FUNCTION_BLOCK FB_IEDClient IMPLEMENTS I_ScsmAbortIndEventSink, I_ScsmGetServerDirectoryCnfEventSink, I_ScsmGetLogicalDeviceDirectoryCnfEventSink, I_ScsmGetLogicalNodeDirectoryCnfEventSink, I_ScsmGetDataValuesCnfEventSink, I_ScsmSetDataValuesCnfEventSink, I_ScsmReportIndEventSink, I_ScsmControlCnfEventSink, I_ScsmLastApplErrorIndEventSink, I_ScsmCommandTerminationIndEventSink
VAR_INPUT
	fbConnection		: FB_iec61850ClientClass := (ipAbortInd:=THIS^, ipGetServerDirectoryCnf:=THIS^, ipGetLogicalDeviceDirectoryCnf:=THIS^, ipGetLogicalNodeDirectoryCnf:=THIS^, ipGetDataValuesCnf:=THIS^, ipSetDataValuesCnf:=THIS^, ipReportInd:=THIS^, ipControlCnf:=THIS^, ipLastApplErrorInd:=THIS^, ipCommandTerminationInd:=THIS^);
END_VAR
VAR
	_bAbort				: BOOL; (* Rising edge activates AbortReq() command execution *)
	_bDisconnect		: BOOL; (* Rising edge activates ReleaseReq() command execution *)
	_bConnect			: BOOL; (* Rising edge activates AssociateReq() command execution *)
	_bReconnect			: BOOL := TRUE; (* TRUE => reconnect automatically *)
	_bReadAllData		: BOOL := TRUE; (* TRUE => read/refresh all data values on reconnect *)
	
	state				: BYTE;
	eState				: E_AsyncEnvironmentState; (* Environment state *)
	bBusy				: BOOL; (* If TRUE => command execution is busy *)
	bSuccess			: BOOL;
	ipResult			: I_AsyncServiceResultClass;
	sLastErrorResult	: T_MaxString;
	fbAbortReason		: FB_ServiceErrorClass := (stError:=SUCCESS_EVENT);
	sLastAbortReason	: T_MaxString;
	nInvokeID			: UDINT;
	eServiceError		: E_AcsiServiceError; (* Latest OnXyzCnf() or OnXyzInd() event handler error *)
	nServiceError		: UDINT; (* Counts OnXyzCnf() and OnXyzInd() event handler errors *)
	nCmdError			: UDINT; (* Counts xyzReq() command errors *)
	sObjReference		: T_AcsiObjectReference; (* DATA object reference *)
	sCtrlReference		: T_AcsiObjectReference; (* CONTROLLABLE-DATA object reference *)
	
	bGetServerDirectory				: BOOL := TRUE; (* Rising edge enumerates logical-devices *)
	bGetLogicalDeviceDirectory		: BOOL := TRUE; (* Rising edge enumerates logical-nodes *)
	bGetLogicalNodeDirectory		: BOOL := TRUE; (* Rising edge enumerates "IEDLD1/LLN0" data-sets *)
	bGetAllServerValues				: BOOL := TRUE; (* Rising edge reads all "IEDLD1" data attribute values *)
	bGetAllDataValues_LLN0_ST		: BOOL := TRUE; (* Rising edge reads all "IEDLD1/LLN0.ST" data attribute values (having selected functional constraint) *)
	bGetDataValues_LLN0_ST_Beh		: BOOL := TRUE; (* Rising edge reads all "IEDLD1/LLN0.ST.Beh" data attribute values (having selected functional constraint) *)

	bGetDataSetValues_LLN0_DS1		: BOOL := TRUE; (* Rising edge reads all member values of data-set: "IEDLD1/LLN0.DS1" *)
	bGetDataSetValues_LLN0_DS2		: BOOL := TRUE; (* Rising edge reads all member values of data-set: "IEDLD1/LLN0.DS2" *)
	bGetDataSetValues_LLN0_DS3		: BOOL := TRUE; (* Rising edge reads all member values of data-set: "IEDLD1/LLN0.DS3" *)
	bGetDataSetValues_LLN0_DS4		: BOOL := TRUE; (* Rising edge reads all member values of data-set: "IEDLD1/LLN0.DS4" *)
	bGetDataSetValues_LLN0_DS5		: BOOL := TRUE; (* Rising edge reads all member values of data-set: "IEDLD1/LLN0.DS5" *)
	bGetDataSetValues_LLN0_DS6		: BOOL := TRUE; (* Rising edge reads all member values of data-set: "IEDLD1/LLN0.DS6" *)
	bGetDataSetValues_LLN0_DS7		: BOOL := TRUE; (* Rising edge reads all member values of data-set: "IEDLD1/LLN0.DS7" *)
	bGetDataSetValues_LLN0_DS8		: BOOL := TRUE; (* Rising edge reads all member values of data-set: "IEDLD1/LLN0.DS8" *)

	bSetDataSetValues_LLN0_DS8		: BOOL := TRUE; (* Rising edge writes all member values of data-set: "IEDLD1/LLN0.DS8" *)
	
	sVendor 						: T_MaxString := 'MyCompany';
	sHwRev							: T_MaxString := '1.0';
	sSwRev 							: T_MaxString := '1.0';
	sSerNum							: T_MaxString := '123456';
	sModel							: T_MaxString := 'My61850Model';
	sLocation						: T_MaxString := 'MyLocation';
	sConfigRev						: T_MaxString := '1';
	nRev							: UDINT:=0;
END_VAR

fbConnection.Execute();
eState:= fbConnection.eState;

CASE state OF
	0: (* Initial state *)
		IF _bAbort THEN (* Abort connection => execute AbortReq() command *)
			_bAbort:= FALSE;
			bSuccess:= fbConnection.AbortReq(ipReason:=fbAbortReason, ipSink:=0, ipResult=>ipResult);
			state:= SEL(bSuccess, 100, 1);
		ELSIF eState = E_AsyncEnvironmentState.Idle AND (_bConnect OR _bReconnect) THEN (* Open/establish connection => execute AssociateReq() command *)
			_bConnect:= FALSE;
			bGetAllServerValues:= SEL(_bReadAllData, bGetAllServerValues, TRUE);
			bSuccess:= fbConnection.AssociateReq(ipSink:=0, ipResult=>ipResult);
			state:= SEL(bSuccess, 100, 1);
		ELSIF eState = E_AsyncEnvironmentState.Established AND _bDisconnect THEN (* Close/release connection => execute ReleaseReq() command *)
			_bDisconnect:= FALSE;
			bSuccess:= fbConnection.ReleaseReq(ipSink:=0, ipResult=>ipResult);
			state:= SEL(bSuccess, 100, 1);
		ELSIF eState = E_AsyncEnvironmentState.Established THEN (* Connection established => exchange IED data *)
			state:= 10;
		END_IF
		_bConnect:= FALSE;
		_bDisconnect:= FALSE;
		(*==================================================================================================================================================================*)
	1: (* Wait for AbortReq() or ReleaseReq() or AssociateReq() command completion *)
		IF ipResult <> 0 THEN
			ipResult.Execute();
			IF NOT (bBusy:=ipResult.IsBusy()) THEN
				state:= SEL(ipResult.IsCompleted(), 100(* failed or aborted *), 0(* succeeded *));
			END_IF
		END_IF
		(*==================================================================================================================================================================*)
	10: (* Read/Write IED data *)
		IF bGetServerDirectory THEN (* Example => execute GetServerDirectoryReq() command *)
			bGetServerDirectory:= FALSE;
			bSuccess:= fbConnection.GetServerDirectoryReq(ipServer:=fbIED, eClass:=E_AcsiServerDirectoryClass.LogicalDevice, hUser:=0, ipSink:=0, nInvokeID=>nInvokeID, ipResult=>ipResult);
			state:= SEL(bSuccess, 100, 11);
		ELSIF bGetLogicalDeviceDirectory THEN (* Example => execute GetLogicalDeviceDirectoryReq() command *)
			bGetLogicalDeviceDirectory:= FALSE;
			bSuccess:= fbConnection.GetLogicalDeviceDirectoryReq(ipLogicalDevice:=fbIED.IEDLD1, hUser:=0, ipSink:=0, nInvokeID=>nInvokeID, ipResult=>ipResult);
			state:= SEL(bSuccess, 100, 11);
		ELSIF bGetLogicalNodeDirectory THEN (* Example => execute GetLogicalNodeDirectoryReq() command *)
			bGetLogicalNodeDirectory:= FALSE;
			bSuccess:= fbConnection.GetLogicalNodeDirectoryReq(ipLogicalNode:=fbIED.IEDLD1.LLN0, eClass:=E_AcsiLogicalNodeClass.DataSet, hUser:=0, ipSink:=0, nInvokeID=>nInvokeID, ipResult=>ipResult);
			state:= SEL(bSuccess, 100, 11);
		ELSIF bGetAllServerValues THEN (* Example => execute GetAllServerValues() command *)
			bGetAllServerValues:= FALSE;
			bSuccess:= fbConnection.GetAllServerValuesReq(ipServer:=fbIED, hUser:=0, ipSink:=0, nInvokeID=>nInvokeID, ipResult=>ipResult);
			state:= SEL(bSuccess, 100, 11);
		ELSIF bGetAllDataValues_LLN0_ST THEN (* Example => execute GetAllDataValuesReq() command *)
			bGetAllDataValues_LLN0_ST:= FALSE;
			bSuccess:= fbConnection.GetAllDataValuesReq(ipLogicalNode:=fbIED.IEDLD1.LLN0, eFc:=E_AcsiFc.ST_, hUser:=0, ipSink:=0, nInvokeID=>nInvokeID, ipResult=>ipResult);
			state:= SEL(bSuccess, 100, 11);
		ELSIF bGetDataValues_LLN0_ST_Beh THEN (* Example => execute GetDataValuesReq() command *)
			bGetDataValues_LLN0_ST_Beh:= FALSE;
			bSuccess:= fbConnection.GetDataValuesReq(ipData:=fbIED.IEDLD1.LLN0.Beh, eFc:=E_AcsiFc.ST_, hUser:=0, ipSink:=0, nInvokeID=>nInvokeID, ipResult=>ipResult);
			state:= SEL(bSuccess, 100, 11);
		(*==================================================================================================================================================================*)
		ELSIF bGetDataSetValues_LLN0_DS1 THEN(* Example => execute GetDataSetValuesReq() command (reads all member values of data-set: "IEDLD1/LLN0.DS1") *)
			bGetDataSetValues_LLN0_DS1:= FALSE;
			bSuccess:= fbConnection.GetDataSetValuesReq(ipDataSet:=fbIED.IEDLD1.LLN0.DS1, hUser:=0, ipSink:=0, nInvokeID=>nInvokeID, ipResult=>ipResult);
			state:= SEL(bSuccess, 100, 11);
		ELSIF bGetDataSetValues_LLN0_DS2 THEN(* Example => execute GetDataSetValuesReq() command (reads all member values of data-set: "IEDLD1/LLN0.DS2") *)
			bGetDataSetValues_LLN0_DS2:= FALSE;
			bSuccess:= fbConnection.GetDataSetValuesReq(ipDataSet:=fbIED.IEDLD1.LLN0.DS2, hUser:=0, ipSink:=0, nInvokeID=>nInvokeID, ipResult=>ipResult);
			state:= SEL(bSuccess, 100, 11);
		ELSIF bGetDataSetValues_LLN0_DS3 THEN(* Example => execute GetDataSetValuesReq() command (reads all member values of data-set: "IEDLD1/LLN0.DS3") *)
			bGetDataSetValues_LLN0_DS3:= FALSE;
			bSuccess:= fbConnection.GetDataSetValuesReq(ipDataSet:=fbIED.IEDLD1.LLN0.DS3, hUser:=0, ipSink:=0, nInvokeID=>nInvokeID, ipResult=>ipResult);
			state:= SEL(bSuccess, 100, 11);
		ELSIF bGetDataSetValues_LLN0_DS4 THEN(* Example => execute GetDataSetValuesReq() command (reads all member values of data-set: "IEDLD1/LLN0.DS4") *)
			bGetDataSetValues_LLN0_DS4:= FALSE;
			bSuccess:= fbConnection.GetDataSetValuesReq(ipDataSet:=fbIED.IEDLD1.LLN0.DS4, hUser:=0, ipSink:=0, nInvokeID=>nInvokeID, ipResult=>ipResult);
			state:= SEL(bSuccess, 100, 11);
		ELSIF bGetDataSetValues_LLN0_DS5 THEN(* Example => execute GetDataSetValuesReq() command (reads all member values of data-set: "IEDLD1/LLN0.DS5") *)
			bGetDataSetValues_LLN0_DS5:= FALSE;
			bSuccess:= fbConnection.GetDataSetValuesReq(ipDataSet:=fbIED.IEDLD1.LLN0.DS5, hUser:=0, ipSink:=0, nInvokeID=>nInvokeID, ipResult=>ipResult);
			state:= SEL(bSuccess, 100, 11);
		ELSIF bGetDataSetValues_LLN0_DS6 THEN(* Example => execute GetDataSetValuesReq() command (reads all member values of data-set: "IEDLD1/LLN0.DS6") *)
			bGetDataSetValues_LLN0_DS6:= FALSE;
			bSuccess:= fbConnection.GetDataSetValuesReq(ipDataSet:=fbIED.IEDLD1.LLN0.DS6, hUser:=0, ipSink:=0, nInvokeID=>nInvokeID, ipResult=>ipResult);
			state:= SEL(bSuccess, 100, 11);
		ELSIF bGetDataSetValues_LLN0_DS7 THEN(* Example => execute GetDataSetValuesReq() command (reads all member values of data-set: "IEDLD1/LLN0.DS7") *)
			bGetDataSetValues_LLN0_DS7:= FALSE;
			bSuccess:= fbConnection.GetDataSetValuesReq(ipDataSet:=fbIED.IEDLD1.LLN0.DS7, hUser:=0, ipSink:=0, nInvokeID=>nInvokeID, ipResult=>ipResult);
			state:= SEL(bSuccess, 100, 11);
		ELSIF bGetDataSetValues_LLN0_DS8 THEN(* Example => execute GetDataSetValuesReq() command (reads all member values of data-set: "IEDLD1/LLN0.DS8") *)
			bGetDataSetValues_LLN0_DS8:= FALSE;
			bSuccess:= fbConnection.GetDataSetValuesReq(ipDataSet:=fbIED.IEDLD1.LLN0.DS8, hUser:=0, ipSink:=0, nInvokeID=>nInvokeID, ipResult=>ipResult);
			state:= SEL(bSuccess, 100, 11);
		ELSIF bSetDataSetValues_LLN0_DS8 THEN(* Example => execute SetDataSetValuesReq() command (writes all member values of data-set: "IEDLD1/LLN0.DS8") *)
			bSetDataSetValues_LLN0_DS8:= FALSE;
			
			(* As example we modify some description data values *)
			sConfigRev:= TO_STRING(nRev:=nRev+1);
			sHwRev:= TO_STRING(TO_REAL(nRev));
			sSwRev:= TO_STRING(TO_REAL(nRev));
			
			fbIED.IEDLD1.LPHD1.PhyNam.Vendor.sValue:= sVendor;
			fbIED.IEDLD1.LPHD1.PhyNam.hwRev.sValue:= sHwRev;
			fbIED.IEDLD1.LPHD1.PhyNam.swRev.sValue:= sSwRev;
			fbIED.IEDLD1.LPHD1.PhyNam.serNum.sValue:= sSerNum;
			fbIED.IEDLD1.LPHD1.PhyNam.model.sValue:= sModel;
			fbIED.IEDLD1.LPHD1.PhyNam.location.sValue:= sLocation;
			
			fbIED.IEDLD1.LLN0.NamPlt.vendor.sValue:= sVendor;
			fbIED.IEDLD1.LLN0.NamPlt.swRev.sValue:= sSwRev;
			fbIED.IEDLD1.LLN0.NamPlt.d.sValue:= 'LLN0 demo node';
			fbIED.IEDLD1.LLN0.NamPlt.configRev.sValue:= sConfigRev;
			
			fbIED.IEDLD1.MMXU1.NamPlt.vendor.sValue:= sVendor;
			fbIED.IEDLD1.MMXU1.NamPlt.swRev.sValue:= sSwRev;
			fbIED.IEDLD1.MMXU1.NamPlt.d.sValue:= 'MMXU1 demo node';
			fbIED.IEDLD1.MMXU1.NamPlt.configRev.sValue:= sConfigRev;

			fbIED.IEDLD1.XCBR1.NamPlt.vendor.sValue:= sVendor;
			fbIED.IEDLD1.XCBR1.NamPlt.swRev.sValue:= sSwRev;
			fbIED.IEDLD1.XCBR1.NamPlt.d.sValue:= 'XCBR1 demo node';
			fbIED.IEDLD1.XCBR1.NamPlt.configRev.sValue:= sConfigRev;

			fbIED.IEDLD1.CSWI1.NamPlt.vendor.sValue:= sVendor;
			fbIED.IEDLD1.CSWI1.NamPlt.swRev.sValue:= sSwRev;
			fbIED.IEDLD1.CSWI1.NamPlt.d.sValue:= 'CSWI1 demo node';
			fbIED.IEDLD1.CSWI1.NamPlt.configRev.sValue:= sConfigRev;

			fbIED.IEDLD1.LEDGGIO1.NamPlt.vendor.sValue:= sVendor;
			fbIED.IEDLD1.LEDGGIO1.NamPlt.swRev.sValue:= sSwRev;
			fbIED.IEDLD1.LEDGGIO1.NamPlt.d.sValue:= 'LEDGGIO1 demo node';
			
			fbIED.IEDLD1.LEDGGIO2.NamPlt.vendor.sValue:= sVendor;
			fbIED.IEDLD1.LEDGGIO2.NamPlt.swRev.sValue:= sSwRev;
			fbIED.IEDLD1.LEDGGIO2.NamPlt.d.sValue:= 'LEDGGIO2 demo node';

			fbIED.IEDLD1.LEDGGIO3.NamPlt.vendor.sValue:= sVendor;
			fbIED.IEDLD1.LEDGGIO3.NamPlt.swRev.sValue:= sSwRev;
			fbIED.IEDLD1.LEDGGIO3.NamPlt.d.sValue:= 'LEDGGIO3 demo node';

			fbIED.IEDLD1.LEDGGIO4.NamPlt.vendor.sValue:= sVendor;
			fbIED.IEDLD1.LEDGGIO4.NamPlt.swRev.sValue:= sSwRev;
			fbIED.IEDLD1.LEDGGIO4.NamPlt.d.sValue:= 'LEDGGIO4 demo node';

			fbIED.IEDLD1.LEDGGIO5.NamPlt.vendor.sValue:= sVendor;
			fbIED.IEDLD1.LEDGGIO5.NamPlt.swRev.sValue:= sSwRev;
			fbIED.IEDLD1.LEDGGIO5.NamPlt.d.sValue:= 'LEDGGIO5 demo node';

			fbIED.IEDLD1.LEDGGIO6.NamPlt.vendor.sValue:= sVendor;
			fbIED.IEDLD1.LEDGGIO6.NamPlt.swRev.sValue:= sSwRev;
			fbIED.IEDLD1.LEDGGIO6.NamPlt.d.sValue:= 'LEDGGIO6 demo node';

			fbIED.IEDLD1.LEDGGIO7.NamPlt.vendor.sValue:= sVendor;
			fbIED.IEDLD1.LEDGGIO7.NamPlt.swRev.sValue:= sSwRev;
			fbIED.IEDLD1.LEDGGIO7.NamPlt.d.sValue:= 'LEDGGIO7 demo node';

			fbIED.IEDLD1.LEDGGIO8.NamPlt.vendor.sValue:= sVendor;
			fbIED.IEDLD1.LEDGGIO8.NamPlt.swRev.sValue:= sSwRev;
			fbIED.IEDLD1.LEDGGIO8.NamPlt.d.sValue:= 'LEDGGIO8 demo node';

			fbIED.IEDLD1.ATCC1.NamPlt.vendor.sValue:= sVendor;
			fbIED.IEDLD1.ATCC1.NamPlt.swRev.sValue:= sSwRev;
			fbIED.IEDLD1.ATCC1.NamPlt.d.sValue:= 'ATCC1 demo node';
			fbIED.IEDLD1.ATCC1.NamPlt.configRev.sValue:= sConfigRev;
			
			bSuccess:= fbConnection.SetDataSetValuesReq(ipDataSet:=fbIED.IEDLD1.LLN0.DS8, hUser:=0, ipSink:=0, nInvokeID=>nInvokeID, ipResult=>ipResult);
			state:= SEL(bSuccess, 100, 11);
		ELSE
			state:= 0;
		END_IF
		(*==================================================================================================================================================================*)
	11: (* Wait for GetServerDirectoryReq(), GetLogicalDeviceDirectoryReq(), GetLogicalNodeDirectoryReq(), GetAllServerValuesReq(), GetAllDataValuesReq(), GetDataValuesReq(), GetDataSetValuesReq() or SetDataSetValuesReq() command completion *)
		IF ipResult <> 0 THEN
			ipResult.Execute();
			IF NOT (bBusy:=ipResult.IsBusy()) THEN
				state:= SEL(ipResult.IsCompleted(), 100(* failed or aborted *), 0(* succeeded *));
			END_IF
		END_IF
		(*==================================================================================================================================================================*)
	100: (* Error state *)
		state:= 0;
		IF ipResult <> 0 THEN
			nCmdError:= nCmdError + 1;
			sLastErrorResult:= ipResult.Dump();
		END_IF
END_CASE

PROPERTY bAbort : BOOL
SET
_bAbort:= bAbort;
END_SET
END_PROPERTY

PROPERTY bConnect : BOOL
SET
_bConnect:= bConnect;
END_SET
END_PROPERTY

PROPERTY bDisconnect : BOOL
SET
_bDisconnect:= bDisconnect;
END_SET
END_PROPERTY

PROPERTY bReconnect : BOOL
SET
_bReconnect:= bReconnect;
END_SET
END_PROPERTY

(* This method receives IEC61850::Abort.ind primitive. *)
METHOD OnAbortInd
VAR_INPUT
	ipAA		: I_ScsmAssociationClass; (* Application association. If = 0 => optional. *)
	bPAbort		: BOOL; (* TRUE => P-Abort.request(), issued by provider, FALSE => Abort.request(), issued by user. *)
	ipReason	: I_ServiceErrorClass; (* Abort reason. *)
	ipData		: I_BaseStreamClass; (* Optional data. If = 0 => default, no data. *)
END_VAR
VAR
END_VAR
IF ipReason <> 0 THEN
	sLastAbortReason:= ipReason.Dump();
END_IF
END_METHOD

(* This method receives buffered IEC61850::Report.ind primitive. *)
METHOD OnBufferedReportInd
VAR_INPUT
	ipAA		: I_ScsmAssociationClass; (* Application association. If = 0 => optional. *)
	info		: ST_ScsmReportEventInfo;
	ipBrcb		: I_AcsiCommonBufferedReportControlBlockClass; (* Interface pointer to BRCB object. *)
	ipDataSet	: I_AcsiCommonDataSetClass; (* Interface pointer to data-set object. *)
	ipData		: I_AcsiCommonDataClass; (* Interface pointer to reported data object. *)
	eFc			: E_AcsiFc; (* Functional constraint of reported data. *)
	eError		: E_AcsiServiceError; (* Data access error code. *)
END_VAR
VAR
END_VAR
IF eError <> E_AcsiServiceError.NoError THEN
	eServiceError:= eError;
	nServiceError:= nServiceError + 1;
END_IF
IF ipData <> 0 THEN
	sObjReference:= ipData.GetObjectReference();
END_IF
END_METHOD

(* This method receives IEC61850::CommandTermination.ind primitive. *)
METHOD OnCommandTerminationInd
VAR_INPUT
	ipAA		: I_ScsmAssociationClass; (* Application association. If = 0 => optional. *)
	info		: ST_ScsmCommandTerminationEventInfo;
	ipCtrl		: I_AcsiCommonControllableDataClass; (* Interface pointer to controllable data object. *)
	ipData		: I_AcsiCommonDataClass; (* Interface pointer to Oper/Cancel/SBO or SBOw data object. *)
	eFc			: E_AcsiFc; (* Functional constraint (CO). *)
	eError		: E_AcsiServiceError; (* Error code. *)
END_VAR
VAR
END_VAR
IF eError <> E_AcsiServiceError.NoError THEN
	eServiceError:= eError;
	nServiceError:= nServiceError + 1;
END_IF
IF ipCtrl <> 0 THEN
	sCtrlReference:= ipCtrl.GetObjectReference();
END_IF
IF ipData <> 0 THEN
	sObjReference:= ipData.GetObjectReference();
END_IF
END_METHOD

(* This method receives IEC61850::Control[Select|Operate|SelectWithValue|Cancel].cnf primitive. *)
METHOD OnControlCnf
VAR_INPUT
	ipAA		: I_ScsmAssociationClass; (* Application association. If = 0 => optional. *)
	info		: ST_ScsmConfirmedEventInfo;
	ipCtrl		: I_AcsiCommonControllableDataClass; (* Interface pointer to controllable data object. *)
	ipData		: I_AcsiCommonDataClass; (* Interface pointer to Oper/Cancel/SBO or SBOw data object. *)
	eFc			: E_AcsiFc; (* Functional constraint (CO). *)
	eError		: E_AcsiServiceError; (* Write/Read data access error code. *)
END_VAR
VAR
END_VAR
IF eError <> E_AcsiServiceError.NoError THEN
	eServiceError:= eError;
	nServiceError:= nServiceError + 1;
END_IF
IF ipCtrl <> 0 THEN
	sCtrlReference:= ipCtrl.GetObjectReference();
END_IF
IF ipData <> 0 THEN
	sObjReference:= ipData.GetObjectReference();
END_IF
END_METHOD

(* This method receives IEC61850::GetDataValues.cnf primitive. *)
METHOD OnGetDataValuesCnf
VAR_INPUT
	ipAA		: I_ScsmAssociationClass; (* Application association. If = 0 => optional. *)
	info		: ST_ScsmConfirmedEventInfo;
	ipData		: I_AcsiCommonDataClass; (* Interface pointer to read data object. *)
	eFc			: E_AcsiFc; (* Functional constraint of read data. *)
	eError		: E_AcsiServiceError; (* Data access error code. *)
END_VAR
VAR
END_VAR
IF eError <> E_AcsiServiceError.NoError THEN
	eServiceError:= eError;
	nServiceError:= nServiceError + 1;
END_IF
IF ipData <> 0 THEN
	sObjReference:= ipData.GetObjectReference();
END_IF
END_METHOD

(* This method receives IEC61850::GetLogicalDeviceDirectory.cnf primitive. *)
METHOD OnGetLogicalDeviceDirectoryCnf
VAR_INPUT
	ipAA				: I_ScsmAssociationClass; (* Application association. If = 0 => optional. *)
	info				: ST_ScsmConfirmedEventInfo;
	ipLogicalDevice		: I_AcsiCommonLogicalDeviceClass; (* Interface pointer to logical-device object. *)
	sObjectReference	: T_AcsiObjectReference;
	eError				: E_AcsiServiceError; (* Logical-device class access error code. *)
END_VAR
VAR
END_VAR
IF eError <> E_AcsiServiceError.NoError THEN
	eServiceError:= eError;
	nServiceError:= nServiceError + 1;
END_IF
sObjReference:= sObjectReference;
END_METHOD

(* This method receives IEC61850::GetLogicalNodeDirectory.cnf primitive. *)
METHOD OnGetLogicalNodeDirectoryCnf
VAR_INPUT
	ipAA				: I_ScsmAssociationClass; (* Application association. If = 0 => optional. *)
	info				: ST_ScsmConfirmedEventInfo;
	ipLogicalNode		: I_AcsiCommonLogicalNodeClass; (* Interface pointer to logical-node object. *)
	eClass				: E_AcsiLogicalNodeClass; (* Logical-node directory class (BRCB, URCB, DATA-SET, ... ). *)
	sObjectReference	: T_AcsiObjectReference;
	eError				: E_AcsiServiceError; (* Logical-node class access error code. *)
END_VAR
VAR
END_VAR
IF eError <> E_AcsiServiceError.NoError THEN
	eServiceError:= eError;
	nServiceError:= nServiceError + 1;
END_IF
sObjReference:= sObjectReference;
END_METHOD

(* This method receives IEC61850::GetServerDirectory.cnf primitive. *)
METHOD OnGetServerDirectoryCnf
VAR_INPUT
	ipAA				: I_ScsmAssociationClass; (* Application association. If = 0 => optional. *)
	info				: ST_ScsmConfirmedEventInfo;
	ipServer			: I_AcsiCommonIntelligentElectronicDeviceClass; (* Interface pointer to server object. *)
	eClass				: E_AcsiServerDirectoryClass; (* Server directory class (logical-device or file). *)
	sObjectReference	: T_AcsiObjectReference;
	eError				: E_AcsiServiceError; (* Server class (logical-device) access error code. *)
END_VAR
VAR
END_VAR
IF eError <> E_AcsiServiceError.NoError THEN
	eServiceError:= eError;
	nServiceError:= nServiceError + 1;
END_IF
sObjReference:= sObjectReference;
END_METHOD

(* This method receives IEC61850::LastApplError.ind primitive. *)
METHOD OnLastApplErrorInd
VAR_INPUT
	ipAA		: I_ScsmAssociationClass; (* Application association. If = 0 => optional. *)
	info		: ST_ScsmAdditionalCauseDiagnosticEventInfo;
	ipCtrl		: I_AcsiCommonControllableDataClass; (* Interface pointer to controllable data object. *)
	eError		: E_AcsiServiceError; (* Error code. *)
END_VAR
VAR
END_VAR
IF eError <> E_AcsiServiceError.NoError THEN
	eServiceError:= eError;
	nServiceError:= nServiceError + 1;
END_IF
IF ipCtrl <> 0 THEN
	sCtrlReference:= ipCtrl.GetObjectReference();
END_IF
END_METHOD

(* This method receives IEC61850::SetDataValues.cnf primitive. *)
METHOD OnSetDataValuesCnf
VAR_INPUT
	ipAA		: I_ScsmAssociationClass; (* Application association. If = 0 => optional. *)
	info		: ST_ScsmConfirmedEventInfo;
	ipData		: I_AcsiCommonDataClass; (* Interface pointer to written data object. *)
	eFc			: E_AcsiFc; (* Functional constraint of written data. *)
	eError		: E_AcsiServiceError; (* Data access error code. *)
END_VAR
VAR
END_VAR
IF eError <> E_AcsiServiceError.NoError THEN
	eServiceError:= eError;
	nServiceError:= nServiceError + 1;
END_IF
IF ipData <> 0 THEN
	sObjReference:= ipData.GetObjectReference();
END_IF
END_METHOD

(* This method receives unbuffered IEC61850::Report.ind primitive. *)
METHOD OnUnbufferedReportInd
VAR_INPUT
	ipAA		: I_ScsmAssociationClass; (* Application association. If = 0 => optional. *)
	info		: ST_ScsmReportEventInfo;
	ipUrcb		: I_AcsiCommonUnbufferedReportControlBlockClass; (* Interface pointer to URCB object. *)
	ipDataSet	: I_AcsiCommonDataSetClass; (* Interface pointer to dataset object. *)
	ipData		: I_AcsiCommonDataClass; (* Interface pointer to reported data object. *)
	eFc			: E_AcsiFc; (* Functional constraint of reported data. *)
	eError		: E_AcsiServiceError; (* Data access error code. *)
END_VAR
VAR
END_VAR
IF eError <> E_AcsiServiceError.NoError THEN
	eServiceError:= eError;
	nServiceError:= nServiceError + 1;
END_IF
IF ipData <> 0 THEN
	sObjReference:= ipData.GetObjectReference();
END_IF
END_METHOD

END_FUNCTION_BLOCK
